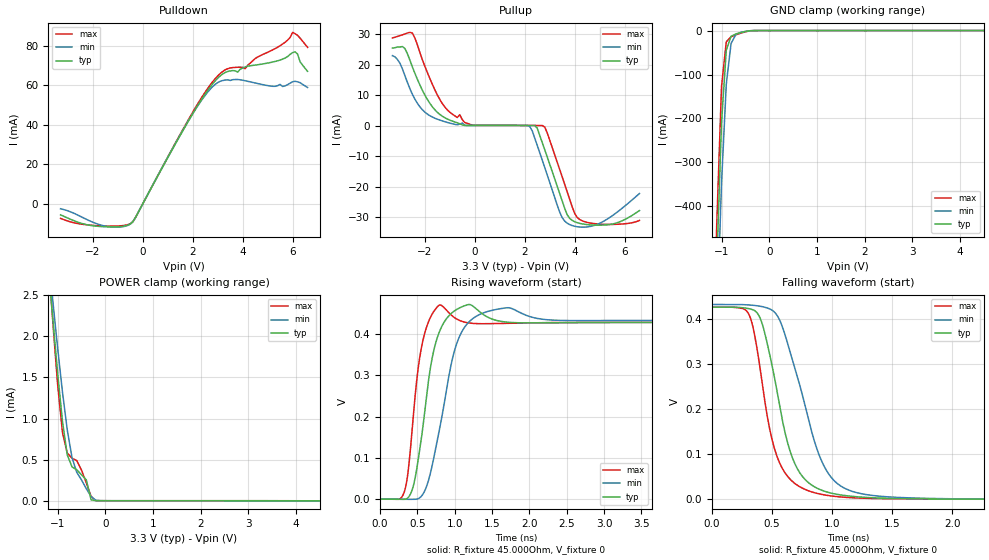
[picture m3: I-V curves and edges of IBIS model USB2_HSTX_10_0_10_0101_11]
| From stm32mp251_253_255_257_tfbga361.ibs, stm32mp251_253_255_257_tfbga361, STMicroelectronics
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[Model] USB2_HSTX_10_0_10_0101_11
Model_type   Output
Polarity   Non-Inverting
Enable   Active-High
C_comp   8.036pF   7.631pF   8.569pF
Vmeas = 200.000mV
Vref = 200.000mV
Rref = 45Ohms
Cref = 0pF
[Model Spec]
Vmeas   200.000mV   200.000mV   200.000mV
Vref   200.000mV   200.000mV   200.000mV
| This model is not intended for timing simulations.
| Warnings about Cref, Vref & Rref can be ignored
[Temperature Range]   25.000   125.000   -40.000
[Voltage Range]   3.300V   3.070V   3.630V
[GND Clamp Reference]   0.00V   0.00V   0.00V
[Pulldown Reference]   0.00V   0.00V   0.00V
[POWER Clamp Reference]   3.300V   3.070V   3.630V
[Pullup Reference]   3.300V   3.070V   3.630V
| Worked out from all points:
|   slope of the pulldown table from 0 to 0.495 V, typ, clamps not added: 42.6 ohm
|   GND clamp passes 1 mA (typ) near -0.43 V on its own axis
|   POWER clamp passes 1 mA (typ) near -0.91 V on its own axis
|   rising waveform, R_fixture 45.000Ohm, V_fixture 0: 20-80 % time 196ps typ, 274ps min, 143ps max; typ from 0 V to 0.428 V
|   falling waveform, R_fixture 45.000Ohm, V_fixture 0: 20-80 % time 216ps typ, 280ps min, 185ps max; typ from 0.427 V to 0 V
[GND Clamp]
-3.3V     -11.02A    -10.62A    -11.32A
-1.2V     -931.6mA   -1.049A    -855.7mA
-1.1V     -533.1mA   -671.7mA   -440.2mA
-1V       -209.4mA   -347mA     -127.3mA
-900mV    -44.44mA   -121.7mA   -25.6mA
-800mV    -13.15mA   -29.48mA   -14.15mA
-700mV    -7.742mA   -9.125mA   -9.769mA
-500mV    -2.127mA   -1.981mA   -2.894mA
-300mV    -19.45uA   -62.22uA   -13.77uA
6.6V      10.37uA    26.59uA    21.05uA
[Power Clamp]
-3.3V     3.206A     2.174A     4.855A
-1.2V     2.88mA     3.008mA    2.969mA
-1.1V     2.195mA    2.419mA    2.156mA
-1V       1.545mA    1.853mA    1.406mA
-900mV    967.6uA    1.324mA    831.4uA
-800mV    558uA      864.5uA    580.3uA
-700mV    412uA      525.9uA    517uA
-600mV    376.6uA    345uA      488.5uA
-400mV    254.2uA    146.6uA    216.8uA
-300mV    11.21uA    52.87uA    53.51uA
-100mV    94.86nA    985nA      361.1nA
6.6V      -2.8uA     -5.18uA    -2.986uA
[Pulldown]
-3.3V     -5.671mA   -2.581mA   -7.449mA
-1.6V     -11.64mA   -11.09mA   -11.31mA
-500mV    -10.25mA   -10.32mA   -10.1mA
1.9V      43.42mA    43.46mA    44.13mA
2.9V      62.15mA    60.37mA    63.26mA
3.4V      66.87mA    62.63mA    68.29mA
4.1V      69.19mA    62.19mA    68.26mA
4.5V      70.11mA    61.06mA    73.4mA
5.6V      73.12mA    59.29mA    80.76mA
6V        76.42mA    61.68mA    86.69mA
6.1V      76.81mA    61.93mA    85.99mA
6.6V      66.95mA    58.79mA    79.1mA
[Pullup]
-3.3V     25.37mA    22.89mA    28.68mA
-2.8V     25.24mA    16.37mA    30mA
-2.5V     19.22mA    10.28mA    30.28mA
-1.7V     6.185mA    2.827mA    13.54mA
-400mV    111.7uA    77.66uA    1.021mA
2.2V      68.64uA    -249uA     104.8uA
2.5V      -770.9uA   -6.355mA   83.47uA
2.8V      -7.785mA   -13.58mA   -409.6uA
3.4V      -22.12mA   -28.2mA    -14.26mA
3.8V      -30.28mA   -32.32mA   -24mA
4.4V      -32.24mA   -33.17mA   -31.39mA
6.6V      -27.75mA   -22.18mA   -30.98mA
[Ramp]
R_load=45.000Ohm
dV/dt_r   628.619mV/1.030ns  596.892mV/1.065ns  682.266mV/960.000ps
dV/dt_f   630.821mV/240.000ps  599.813mV/315.000ps  684.093mV/215.000ps
[Rising waveform]
R_fixture=45.000Ohm
V_fixture=0
0s        452.1nV    3.134uV    468nV
310ps     -466.1uV   -354.1uV   11.02mV
430ps     22.58mV    -459.5uV   168.2mV
570ps     169.8mV    10.84mV    381mV
680ps     324mV      67.14mV    442mV
800ps     407.5mV    172.8mV    470mV
960ps     450.6mV    332.8mV    444.6mV
1.09ns    465.2mV    403.6mV    430.8mV
1.62ns    430.3mV    461.3mV    425.4mV
9.9ns     427.9mV    433.7mV    427.8mV
[Falling waveform]
R_fixture=45.000Ohm
V_fixture=0
0s        427.4mV    433.2mV    427.3mV
310ps     423.7mV    432.1mV    409.5mV
410ps     396.3mV    428.9mV    273mV
540ps     241.5mV    409.4mV    95.91mV
620ps     134.7mV    354.7mV    54.11mV
700ps     73.11mV    281.9mV    33.13mV
950ps     16.78mV    65.04mV    9.087mV
1.18ns    6.256mV    16.58mV    3.314mV
1.74ns    997.4uV    2.488mV    744.9uV
9.9ns     14.09uV    31.29uV    4.153uV
